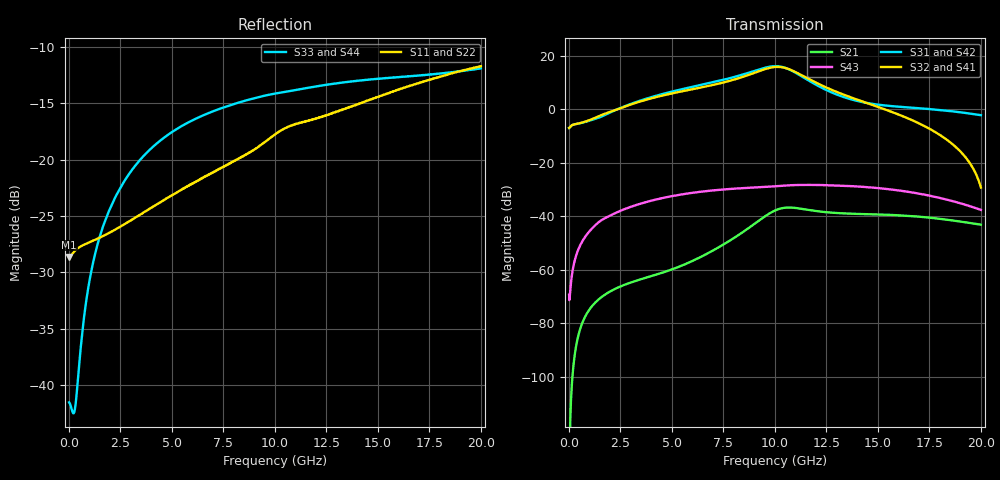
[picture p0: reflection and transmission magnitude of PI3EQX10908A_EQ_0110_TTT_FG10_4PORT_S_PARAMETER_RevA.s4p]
! NPort=4 DATA=2000 NOISE=0 GROUPDELAY=0 COMPLEX_DATAFORMAT=POLAR
! NumOfBlock=1 NumOfParam=0
! .MODEL Smodel S TSTONEFILE=PI3EQX10908A_EQ_0110_TTT_FG10_4PORT_S_PARAMETER_RevA.s4p TYPE=S
!  -- The above .MODEL line can be used for the S element in the netlist.
! The s parameter is extracted from the linear redriver, it is not bi-directional; only s(4,1)s(4,2) and s(3,1)s(3,2)
! should be the insertion loss
!Port definition:
!Port1 = input+
!Port2 = input-
!Port3 = output+
!Port4 = output-
# Hz S MA R  50
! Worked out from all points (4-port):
!   2000 points, 10 MHz to 20 GHz, reference 50 ohm
!   strongest paths, dB at 10 MHz, 5.01 GHz, 10.01 GHz, 15.01 GHz, 20 GHz:
!     S32: -6.9, 6.0, 15.9, 0.9, -29.2
!     S41: -6.9, 6.0, 15.9, 0.9, -29.2
!     S31: -6.9, 6.7, 16.2, 1.8, -2.1
!     S42: -6.9, 6.7, 16.2, 1.8, -2.1
!     S43: -69.4, -32.4, -28.7, -29.4, -37.6
!     S21: -127.2, -59.9, -37.8, -39.3, -43.1
!   lowest |S11| = -28.6 dB at 10 MHz (marker M1), VSWR 1.08, Z = 46.4 - j0.024 ohm
!   |S11| at or under -10 dB: start of sweep to end of sweep
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1e7  0.03701 -179.6  4.342e-07 14.4  0 0.0  0 0.0
     4.342e-07 14.4  0.03701 -179.6  0 0.0  0 0.0
     0.451 1.0  0.451 -179.0  0.008374 26.0  0.00034 -27.1
     0.451 -179.0  0.451 1.0  0.00034 -27.1  0.008374 26.0
7.45e9  0.09226 -118.0  0.002882 133.6  7.543e-07 55.5  3.419e-07 133.0
        0.002881 133.6  0.0923 -117.9  3.419e-07 133.0  7.543e-07 55.5
        3.553 -55.5  3.167 117.9  0.1696 6.0  0.03166 8.8
        3.167 117.9  3.553 -55.5  0.03166 8.8  0.1696 6.0
9.48e9  0.1189 -111.0  0.009733 114.0  3.461e-06 12.0  2.158e-06 118.4
        0.009733 114.0  0.1189 -111.0  2.158e-06 118.4  3.461e-06 12.0
        5.994 -111.7  5.626 62.9  0.1918 -9.1  0.03538 -11.5
        5.626 62.9  5.994 -111.7  0.03538 -11.5  0.1918 -9.1
1.048e10  0.1378 -111.6  0.01446 76.0  4.934e-06 -22.1  5.341e-06 82.1
          0.01446 76.0  0.1379 -111.6  5.341e-06 82.1  4.934e-06 -22.1
          6.053 -162.2  6.016 11.0  0.1997 -15.8  0.03766 -21.7
          6.016 11.0  6.053 -162.2  0.03766 -21.7  0.1997 -15.8
1.148e10  0.1472 -113.1  0.01344 44.4  5.19e-06 -30.8  8.264e-06 45.2
          0.01344 44.4  0.1472 -113.1  8.264e-06 45.2  5.19e-06 -30.8
          3.788 158.6  4.022 -32.1  0.2074 -21.6  0.03869 -34.3
          4.022 -32.1  3.788 158.6  0.03869 -34.3  0.2074 -21.6
1.364e10  0.1712 -111.5  0.0112 15.4  1.379e-05 -37.7  1.695e-05 -4.6
          0.0112 15.4  0.1713 -111.5  1.695e-05 -4.6  1.378e-05 -37.7
          1.57 131.4  1.713 -79.2  0.2217 -32.6  0.03682 -60.5
          1.713 -79.2  1.57 131.4  0.03682 -60.5  0.2217 -32.6
2e10  0.2597 -114.4  0.006967 -41.7  9.042e-05 -147.7  7.23e-05 -137.8
      0.006966 -41.7  0.2598 -114.4  7.23e-05 -137.8  9.041e-05 -147.8
      0.782 58.0  0.03456 176.3  0.2539 -52.2  0.01316 -136.7
      0.03456 176.4  0.782 57.9  0.01316 -136.7  0.2539 -52.2
